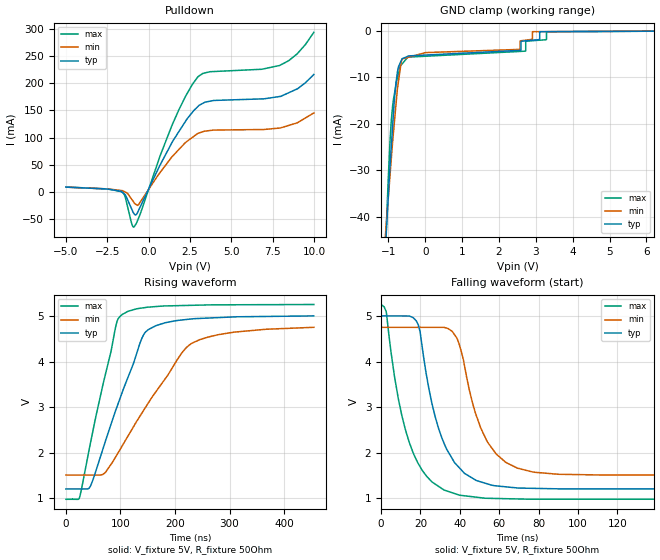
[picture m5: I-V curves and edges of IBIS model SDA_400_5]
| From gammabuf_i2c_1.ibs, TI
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|   Input/Output open drain SDA_400 model 5V with 400 kHz CLOCK
[Model]   SDA_400_5
Model_type   I/O_open_drain
Vinl = 1.5
Vinh = 3.5
Vmeas = 2.5
Vref = 2.5
Cref = 15pF
Rref = 50
|Signals   SDA
| variable   typ   min   max
|C_comp Average
C_comp   6.7058138e-11   4.6889634e-11   1.0192905e-10
|C_comp Output Low
|C_comp   1.3233200e-10   9.1871810e-11   2.0224130e-10
|C_comp Output High
|C_comp   1.7842760e-12   1.9074570e-12   1.6167470e-12
[Voltage Range]   5   4.75   5.25
[Temperature Range]   27   85   -40
[Pullup Reference]   5   4.75   5.25
[Pulldown Reference]   0   0   0
[Power Clamp Reference]   5   4.75   5.25
[GND Clamp Reference]   -0   0   0
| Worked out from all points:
|   slope of the pulldown table from 0 to 0.75 V, typ, clamps not added: 15.7 ohm
|   falling waveform, V_fixture 5V, R_fixture 50Ohm: 20-80 % time 13.7ns typ, 13.9ns min, 13.6ns max; typ from 5 V to 1.21 V
|   rising waveform, V_fixture 5V, R_fixture 50Ohm: 20-80 % time 66.8ns typ, 104ns min, 46.7ns max; typ from 1.21 V to 5 V
[Pulldown]
|   Voltage   I(typ)   I(min)   I(max)
-5V       8.33mA     8.229mA    8.568mA
-1.637V   7.48uA     2.021mA    -146.3uA
-1.426V   -5.442mA   -676.3uA   -8.669mA
-1.044V   -30.97mA   -13.28mA   -57.16mA
-897.2mV  -40.15mA   -19.65mA   -65.67mA
-618.4mV  -35.24mA   -24.34mA   -49.57mA
1.429V    91.77mA    64.97mA    123.8mA
2.962V    156.8mA    107.4mA    211.6mA
3.936V    168.5mA    113.7mA    221.9mA
7.892V    175.7mA    117.4mA    232.9mA
8.97V     189.7mA    127mA      254.5mA
9.985V    216.4mA    145.4mA    294.4mA
[GND Clamp]
|   Voltage   I(typ)   I(min)   I(max)
-5V       -668.6mA   -488.5mA   -1.015A
-1.057V   -43.47mA   -41.55mA   -42.51mA
-952.4mV  -28.72mA   -30.73mA   -23.22mA
-869.6mV  -18.59mA   -22.52mA   -15.2mA
-751.9mV  -8.782mA   -12.31mA   -10.05mA
-653.5mV  -6.501mA   -6.808mA   -7.4mA
-449.2mV  -5.455mA   -5.735mA   -5.713mA
2.564V    -4.266mA   -4.058mA   -4.498mA
2.603V    -2.296mA   -2.194mA   -4.482mA
2.913V    -2.08mA    -251.5uA   -2.191mA
3.294V    -250.8uA   -237.9uA   -258.6uA
9.985V    0A         0A         0A
[POWER Clamp]
|   Voltage   I(typ)   I(min)   I(max)
-5V       0A         0A         0A
0V        0A         0A         0A
10V       0A         0A         0A
[Ramp]
R_load = 50
|   typ   min   max
dV/dt_r   2.27599/6.67224e-008   1.94313/1.03909e-007   2.56172/4.67982e-008
dV/dt_f   2.27599/1.3533e-008   1.94313/1.36897e-008   2.56172/1.35227e-008
[Falling Waveform]
V_fixture = 5V
V_fixture_min = 4.75V
V_fixture_max = 5.25V
R_fixture = 50Ohm
C_fixture = 0F
|   Time   V(typ)   V(min)   V(max)
0s        5V         4.75V      5.25V
2.597ns   5V         4.75V      5.098V
8.774ns   4.999V     4.75V      3.186V
16.3ns    4.963V     4.75V      2V
19.81ns   4.658V     4.75V      1.696V
29.08ns   2.553V     4.75V      1.269V
39.81ns   1.669V     4.362V     1.072V
54.2ns    1.316V     2.226V     1.003V
77.47ns   1.221V     1.577V     982.6mV
454.6ns   1.207V     1.511V     980.5mV
[Rising Waveform]
V_fixture = 5V
V_fixture_min = 4.75V
V_fixture_max = 5.25V
R_fixture = 50Ohm
C_fixture = 0F
|   Time   V(typ)   V(min)   V(max)
0s        1.207V     1.511V     980.5mV
25.21ns   1.207V     1.512V     1.027V
45.66ns   1.286V     1.512V     2.252V
67.49ns   2.07V      1.524V     3.472V
91.73ns   2.944V     1.919V     4.789V
102.4ns   3.298V     2.135V     5.024V
146.3ns   4.652V     3.002V     5.185V
229.2ns   4.932V     4.388V     5.232V
305.6ns   4.977V     4.639V     5.244V
454.6ns   5V         4.75V      5.25V
